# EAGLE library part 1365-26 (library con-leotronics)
DUAL ROW STRAIGHT HEADER 1364 SERIES. 1.27mm x 1.27mm. Without Fixing Post. SMT Source: http://www.leotronics.co.uk/Conexcon/Data%20Sheets/sec.%20A/1364ing.pdf
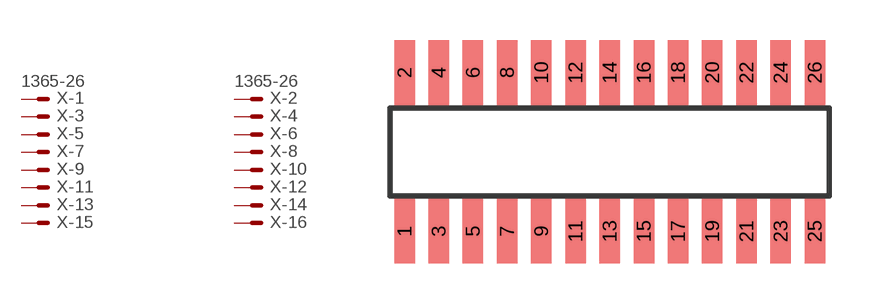
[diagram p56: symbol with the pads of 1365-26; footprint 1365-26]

Designator prefix X; gates -1=MVAL -2=MVAL -3=M -4=M -5=M -6=M -7=M -8=M -9=M -10=M -11=M -12=M -13=M -14=M -15=M -16=M -17=M -18=M -19=M -20=M -21=M -22=M -23=M -24=M -25=M -26=M

## 1365-26 (OC_FARNELL: unknown; OC_NEWARK: unknown)  [1365-26]
1  -1:S  pas
2  -2:S  pas
3  -3:S  pas
4  -4:S  pas
5  -5:S  pas
6  -6:S  pas
7  -7:S  pas
8  -8:S  pas
9  -9:S  pas
10  -10:S  pas
11  -11:S  pas
12  -12:S  pas
13  -13:S  pas
14  -14:S  pas
15  -15:S  pas
16  -16:S  pas
17  -17:S  pas
18  -18:S  pas
19  -19:S  pas
20  -20:S  pas
21  -21:S  pas
22  -22:S  pas
23  -23:S  pas
24  -24:S  pas
25  -25:S  pas
26  -26:S  pas

## Footprint 1365-26 (pad centres in mm)
DUAL ROW STRAIGHT HEADER 1364 SERIES. 1.27mm x 1.27mm. Without Fixing Post. SMT Source: http://www.leotronics.co.uk/Conexcon/Data%20Sheets/sec.%20A/1364ing.pdf
smd 0.76 x 2.4: 1 -7.62,-2.95; 2 -7.62,2.95; 3 -6.35,-2.95; 4 -6.35,2.95; 5 -5.08,-2.95; 6 -5.08,2.95; 7 -3.81,-2.95; 8 -3.81,2.95; 9 -2.54,-2.95; 10 -2.54,2.95; 11 -1.27,-2.95; 12 -1.27,2.95; 13 0,-2.95; 14 0,2.95; 15 1.27,-2.95; 16 1.27,2.95; 17 2.54,-2.95; 18 2.54,2.95; 19 3.81,-2.95; 20 3.81,2.95; 21 5.08,-2.95; 22 5.08,2.95; 23 6.35,-2.95; 24 6.35,2.95; 25 7.62,-2.95; 26 7.62,2.95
